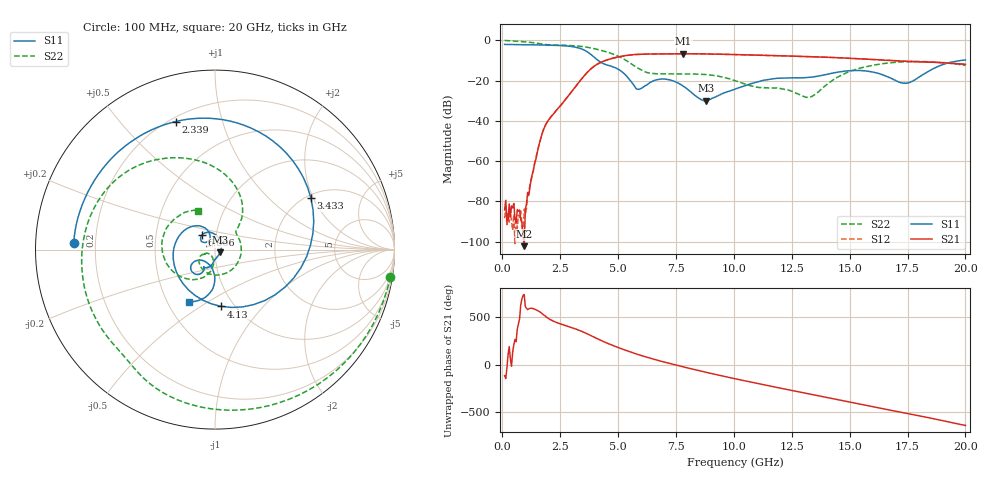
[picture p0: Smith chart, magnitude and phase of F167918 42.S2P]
!  2-Port S-parameters saved by WinCal
! VAR MeasName=S-Parameters (CALIBRATED_DATA) read from VNA (N5242A)
! VAR MeasDate=2016-11-22 10:26:47
! VAR NAME=F167918 42
! VAR FILENAME=F167918 42.S2P
! VAR DATE=2016-11-22 10:26:47
! VAR PHYS_PORTS=1,2
# Hz S DB R 50
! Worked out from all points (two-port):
!   401 points, 100 MHz to 20 GHz, reference 50 ohm
!   highest |S21| = -6.68 dB at 7.811 GHz (marker M1); lowest = -102.2 dB at 945.8 MHz (marker M2)
!   |S21| within 3 dB of the highest: 4.546 GHz to 16.25 GHz (11.7 GHz wide, 113 % of centre)
!   lowest |S11| = -30.0 dB at 8.806 GHz (marker M3), VSWR 1.06, Z = 52.9 - j1.53 ohm
!   |S11| at or under -10 dB: 4.136 GHz to 19.85 GHz (15.72 GHz wide, 131 % of centre)
!   |S22| runs from -28.3 to -0.1 dB; largest |S21 - S12| = 0.0059
!   S11 on the Smith chart (normalised r, x): 100 MHz: 0.12, +0.02; 2.339 GHz: 0.22, +0.71; 3.433 GHz: 2.12, +1.91; 4.13 GHz: 0.87, -0.61; 6.866 GHz: 0.86, +0.14; 20 GHz: 0.64, -0.42
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1e8  -2.07 177.3  -84.20 -117.6  -88.36 99.7  -0.10 -8.8
9.4575e8  -2.19 154.6  -102.21 20.2  -83.82 -115.7  -0.77 -74.3
1.14475e9  -2.23 149.0  -76.98 -130.7  -75.80 -104.1  -0.98 -88.0
1.74175e9  -2.35 130.4  -45.61 173.9  -45.61 173.8  -1.95 -124.4
2.33875e9  -2.54 107.1  -34.76 85.2  -34.73 84.8  -2.31 -152.2
2.93575e9  -3.02 73.3  -26.37 35.9  -26.38 35.8  -2.63 179.3
3.43325e9  -4.35 28.1  -19.06 -9.0  -19.08 -8.9  -3.09 155.2
4.12975e9  -9.94 -83.7  -11.69 -89.2  -11.65 -89.3  -4.61 120.7
4.5775e9  -12.44 -166.7  -9.57 -138.3  -9.53 -138.6  -6.05 99.2
5.22425e9  -16.16 122.3  -7.80 160.6  -7.80 160.3  -9.20 67.7
5.871e9  -24.30 129.4  -7.01 105.8  -7.01 105.7  -13.91 46.6
6.7665e9  -19.34 134.8  -6.79 41.6  -6.80 41.4  -16.69 30.5
6.866e9  -19.21 130.4  -6.78 35.1  -6.81 34.8  -16.68 26.4
7.81125e9  -22.74 77.8  -6.68 -23.9  -6.71 -23.9  -16.73 -30.1
8.80625e9  -30.04 -27.3  -6.79 -81.7  -6.79 -81.8  -17.01 -96.8
1.005e10  -24.24 -93.9  -7.10 -149.3  -7.11 -149.2  -20.08 -151.4
1.189075e10  -18.86 -116.6  -7.68 116.9  -7.66 117.0  -23.79 -155.5
1.338325e10  -18.29 -120.2  -8.17 42.9  -8.13 43.1  -27.83 -117.5
1.53235e10  -15.01 -134.6  -9.13 -52.2  -9.11 -52.4  -14.25 -121.5
1.67165e10  -18.54 -149.2  -9.97 -119.4  -10.02 -119.3  -11.25 -159.1
1.75125e10  -21.29 -115.5  -10.49 -157.4  -10.44 -157.4  -10.63 179.2
2e10  -9.74 -116.4  -11.96 77.2  -11.85 76.9  -12.50 113.6
